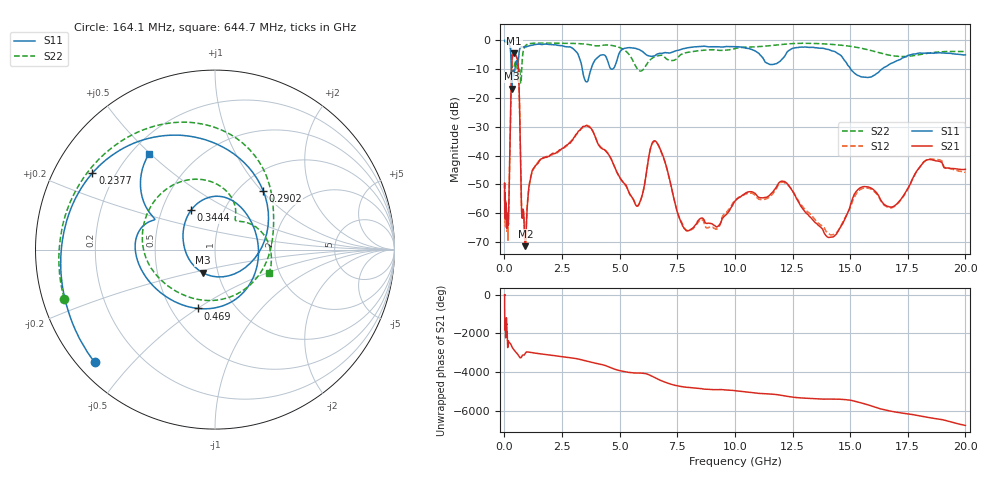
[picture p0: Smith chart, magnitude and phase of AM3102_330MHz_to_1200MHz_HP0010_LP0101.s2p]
! Date/Time: Tue, Sep 11, 2018 5:10 PM
! Network Analyzer: Agilent Technologies E8362B Rev: A.07.50.63
! Sweep from 0.010 to 20.000 GHz, 1601 Points, Sweep Type: LOG
! Power Supply: 4.950 V, 0.001 A
# Hz S DB R 50
!freq MagS11 AngS11 MagS21 AngS21 MagS12 AngS12 MagS22 AngS22
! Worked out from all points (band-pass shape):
!   1601 points, 10 MHz to 20 GHz, reference 50 ohm
!   highest |S21| = -4.40 dB at 416.5 MHz (marker M1); lowest = -71.4 dB at 912 MHz (marker M2)
!   |S21| within 3 dB of the highest: 325.1 MHz to 586 MHz (260.8 MHz wide, 57.3 % of centre)
!   lowest |S11| = -16.7 dB at 319.2 MHz (marker M3), VSWR 1.34, Z = 42.2 - j11.1 ohm
!   |S11| at or under -10 dB: 297.6 MHz to 454.4 MHz (156.8 MHz wide, 41.7 % of centre); 3.379 GHz to 3.761 GHz (382.2 MHz wide, 10.7 % of centre); 15.03 GHz to 16.37 GHz (1.345 GHz wide, 8.57 % of centre)
!   |S22| runs from -14.8 to -0.2 dB; largest |S21 - S12| = 0.011
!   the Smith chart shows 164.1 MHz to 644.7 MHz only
!   S11 on the Smith chart (normalised r, x): 164.1 MHz: 0.05, -0.39; 237.7 MHz: 0.12, +0.28; 290.2 MHz: 1.28, +1.02; 344.4 MHz: 0.70, +0.33; 469 MHz: 0.67, -0.50; 644.7 MHz: 0.27, +0.50
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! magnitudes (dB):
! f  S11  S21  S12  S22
! 10 MHz  0.0  -51.3  -49.7  -0.2
! 35.55 MHz  0.0  -61.0  -60.9  -0.4
! 126.4 MHz  -0.4  -62.9  -62.9  -0.9
! 164.1 MHz  -0.7  -63.4  -66.4  -1.1
! 237.7 MHz  -1.9  -39.0  -39.0  -1.8
! 290.2 MHz  -7.5  -15.9  -16.0  -3.9
! 319.2 MHz  -16.7  -8.2  -8.2  -7.6
! 344.4 MHz  -11.8  -5.9  -6.0  -10.3
! 416.5 MHz  -12.2  -4.4  -4.4  -9.5
! 447.2 MHz  -10.4  -4.6  -4.6  -8.1
! 469 MHz  -9.3  -4.8  -4.8  -7.6
! 644.7 MHz  -3.8  -18.3  -18.4  -9.6
! 750.6 MHz  -2.2  -59.9  -59.5  -10.3
! 912 MHz  -2.3  -71.4  -71.2  -1.8
! 1.59 GHz  -1.4  -41.1  -41.2  -0.9
! 3.634 GHz  -13.8  -29.8  -29.6  -1.4
! 5.652 GHz  -2.7  -56.2  -56.3  -8.2
! 6.58 GHz  -5.0  -35.1  -35.3  -5.5
! 7.882 GHz  -2.7  -66.0  -65.7  -4.2
! 12.09 GHz  -6.1  -48.9  -49.2  -1.3
! 14.14 GHz  -3.4  -68.3  -67.4  -1.3
! 20 GHz  -5.0  -44.8  -45.8  -3.8
